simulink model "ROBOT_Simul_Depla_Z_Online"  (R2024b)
settings: Solver=ode15s  StartTime=0.0  StopTime=0.2  RelTol=1e-3  EnableMultiTasking=on
undefined symbols (not defined in the file): BATI1_Défaut_sldprt, BATI2_Défaut_sldprt, BATI3_Défaut_sldprt, BIELLE_Défaut_sldprt, BRAS_Défaut_sldprt, deg, Drive, EFFECTEUR_Défaut_sldprt, Fichiers, Fichiers_Matlab_sujetB, JOINT_Défaut_sldprt, kg, m, MANETTE_Défaut_sldprt, MATLAB, Matlab, mm, N, PIED_Défaut_sldprt, rad, s, STL, X, Y, Z
libraries: sm_lib x139, fl_lib x42, nesl_utility x19, slpidlib x3
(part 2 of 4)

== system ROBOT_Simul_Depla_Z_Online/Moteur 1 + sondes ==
  In1 : Inport
  Moteur à courant continu1 : Subsystem
  Reference electrique : fl_lib/Electrical/Electrical Elements/Electrical Reference
  Simulink-PS Converter1 : nesl_utility/Simulink-PS Converter  PhysicalDomain=network_engine_domain  SubClassName=ps_input  LeftPortType=input  RightPortType=output  PseudoPeriodic=off  Frequencies=[]  NoiseDistribution=none  NoiseParameters=[]  Unit=V  AffineConversion=off  FilteringAndDerivatives=zero  SimscapeFilterOrder=2  InputFilterTimeConstant=1e-4  UdotUserProvided=1
  Sondes électriques1 : Subsystem
  Source de tension controlée1 : fl_lib/Electrical/Electrical Sources/Controlled Voltage Source
  Conn1 : PMIOPort  Side=Right
  Conn2 : PMIOPort  Port=2  Side=Right
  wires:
  In1/1 -> Simulink-PS Converter1/1
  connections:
  Conn2/RConn1 -- Moteur à courant continu1/RConn2
  Conn1/RConn1 -- Moteur à courant continu1/RConn1
  Source de tension controlée1/LConn1 -- Sondes électriques1/LConn1
  Simulink-PS Converter1/RConn1 -- Source de tension controlée1/RConn1
  Sondes électriques1/RConn2 -- Source de tension controlée1/RConn2 -- Reference electrique/LConn1 -- Moteur à courant continu1/LConn2
  Sondes électriques1/RConn1 -- Moteur à courant continu1/LConn1

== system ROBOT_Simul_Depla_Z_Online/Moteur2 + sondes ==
  In1 : Inport
  Moteur à courant continu2 : Subsystem
  Reference electrique : fl_lib/Electrical/Electrical Elements/Electrical Reference
  Simulink-PS Converter1 : nesl_utility/Simulink-PS Converter  PhysicalDomain=network_engine_domain  SubClassName=ps_input  LeftPortType=input  RightPortType=output  PseudoPeriodic=off  Frequencies=[]  NoiseDistribution=none  NoiseParameters=[]  Unit=V  AffineConversion=off  FilteringAndDerivatives=zero  SimscapeFilterOrder=2  InputFilterTimeConstant=1e-4  UdotUserProvided=1
  Sondes électriques : Subsystem
  Source de tension controlée : fl_lib/Electrical/Electrical Sources/Controlled Voltage Source
  Conn1 : PMIOPort  Side=Right
  Conn2 : PMIOPort  Port=2  Side=Right
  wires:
  In1/1 -> Simulink-PS Converter1/1
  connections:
  Sondes électriques/RConn1 -- Moteur à courant continu2/LConn1
  Source de tension controlée/RConn2 -- Reference electrique/LConn1 -- Sondes électriques/RConn2 -- Moteur à courant continu2/LConn2
  Simulink-PS Converter1/RConn1 -- Source de tension controlée/RConn1
  Source de tension controlée/LConn1 -- Sondes électriques/LConn1
  Conn1/RConn1 -- Moteur à courant continu2/RConn1
  Conn2/RConn1 -- Moteur à courant continu2/RConn2

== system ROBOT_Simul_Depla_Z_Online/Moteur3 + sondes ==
  In1 : Inport
  Moteur à courant continu3 : Subsystem
  Reference electrique : fl_lib/Electrical/Electrical Elements/Electrical Reference
  Simulink-PS Converter1 : nesl_utility/Simulink-PS Converter  PhysicalDomain=network_engine_domain  SubClassName=ps_input  LeftPortType=input  RightPortType=output  PseudoPeriodic=off  Frequencies=[]  NoiseDistribution=none  NoiseParameters=[]  Unit=V  AffineConversion=off  FilteringAndDerivatives=zero  SimscapeFilterOrder=2  InputFilterTimeConstant=1e-4  UdotUserProvided=1
  Sondes électriques3 : Subsystem
  Source de tension controlée3 : fl_lib/Electrical/Electrical Sources/Controlled Voltage Source
  Conn1 : PMIOPort  Side=Right
  Conn2 : PMIOPort  Port=2  Side=Right
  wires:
  In1/1 -> Simulink-PS Converter1/1
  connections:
  Sondes électriques3/RConn1 -- Moteur à courant continu3/LConn1
  Moteur à courant continu3/LConn2 -- Reference electrique/LConn1 -- Source de tension controlée3/RConn2 -- Sondes électriques3/RConn2
  Simulink-PS Converter1/RConn1 -- Source de tension controlée3/RConn1
  Source de tension controlée3/LConn1 -- Sondes électriques3/LConn1
  Conn1/RConn1 -- Moteur à courant continu3/RConn1
  Conn2/RConn1 -- Moteur à courant continu3/RConn2

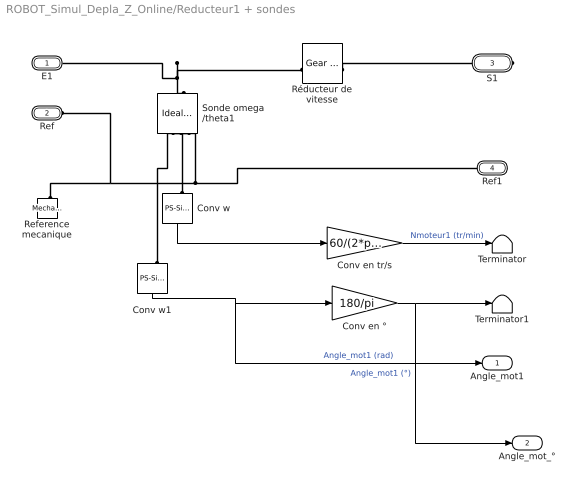
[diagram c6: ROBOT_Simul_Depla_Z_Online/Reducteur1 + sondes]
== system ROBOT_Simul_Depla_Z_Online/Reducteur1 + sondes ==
  Conv en tr/s : Gain  Gain=60/(2*pi)
  Conv en ° : Gain  Gain=180/pi
  Conv w : nesl_utility/PS-Simulink Converter  PhysicalDomain=network_engine_domain  SubClassName=ps_output  LeftPortType=input  RightPortType=output  PseudoPeriodic=off  Frequencies=[]  VectorFormat=1-D array  Unit=1  AffineConversion=off
  Conv w1 : nesl_utility/PS-Simulink Converter  PhysicalDomain=network_engine_domain  SubClassName=ps_output  LeftPortType=input  RightPortType=output  PseudoPeriodic=off  Frequencies=[]  VectorFormat=1-D array  Unit=1  AffineConversion=off
  Reference mecanique : fl_lib/Mechanical/Rotational Elements/Mechanical Rotational Reference
  Réducteur de vitesse : fl_lib/Mechanical/Mechanisms/Gear Box  ratio=7.627  t_in_specify=off  t_in_priority=None  t_in=0 N*m  t_in_nominal_specify=off  t_in_nominal_value=1  t_in_nominal_unit=N*m  t_out_specify=off  t_out_priority=None  t_out=0 N*m  t_out_nominal_specify=off  t_out_nominal_value=1  t_out_nominal_unit=N*m
  Sonde omega /theta1 : fl_lib/Mechanical/Mechanical Sensors/Ideal Rotational Motion Sensor  reference=foundation.enum.MeasurementReference.difference  acceleration_port=false  velocity_port=true  position_port=true  wrap_angle=false  offset=0 rad
  Terminator : Terminator
  Terminator1 : Terminator
  E1 : PMIOPort  Side=Left
  Ref : PMIOPort  Port=2  Side=Left
  S1 : PMIOPort  Port=3  Side=Right
  Ref1 : PMIOPort  Port=4  Side=Right
  Angle_mot1 : Outport  VectorParamsAs1DForOutWhenUnconnected=off
  Angle_mot_° : Outport  Port=2  VectorParamsAs1DForOutWhenUnconnected=off
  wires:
  Conv w1/1 -> Angle_mot1/1, Conv en °/1  "Angle_mot1 (rad)"
  Conv en °/1 -> Angle_mot_°/1, Terminator1/1  "Angle_mot1 (°)"
  Conv w/1 -> Conv en tr/s/1
  Conv en tr/s/1 -> Terminator/1  "Nmoteur1 (tr/min)"
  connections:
  Sonde omega /theta1/LConn1 -- E1/RConn1 -- Réducteur de vitesse/LConn1
  Reference mecanique/LConn1 -- Ref/RConn1 -- Sonde omega /theta1/RConn1 -- Ref1/RConn1
  Conv w/LConn1 -- Sonde omega /theta1/RConn2
  Conv w1/LConn1 -- Sonde omega /theta1/RConn3
  Réducteur de vitesse/RConn1 -- S1/RConn1

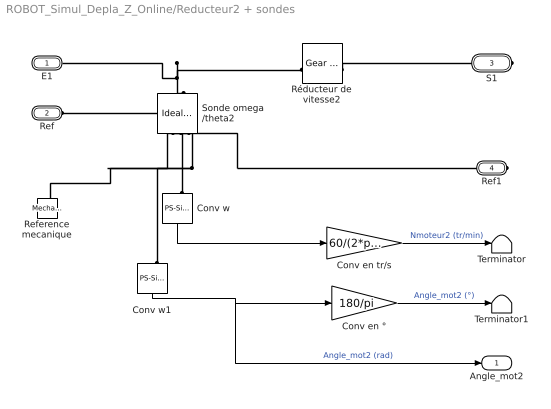
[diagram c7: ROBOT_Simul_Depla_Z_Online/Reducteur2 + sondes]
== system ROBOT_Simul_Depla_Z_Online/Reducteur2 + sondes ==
  Conv en tr/s : Gain  Gain=60/(2*pi)
  Conv en ° : Gain  Gain=180/pi
  Conv w : nesl_utility/PS-Simulink Converter  PhysicalDomain=network_engine_domain  SubClassName=ps_output  LeftPortType=input  RightPortType=output  PseudoPeriodic=off  Frequencies=[]  VectorFormat=1-D array  Unit=1  AffineConversion=off
  Conv w1 : nesl_utility/PS-Simulink Converter  PhysicalDomain=network_engine_domain  SubClassName=ps_output  LeftPortType=input  RightPortType=output  PseudoPeriodic=off  Frequencies=[]  VectorFormat=1-D array  Unit=1  AffineConversion=off
  Reference mecanique : fl_lib/Mechanical/Rotational Elements/Mechanical Rotational Reference
  Réducteur de vitesse2 : fl_lib/Mechanical/Mechanisms/Gear Box  ratio=7.627  t_in_specify=off  t_in_priority=None  t_in=0 N*m  t_in_nominal_specify=off  t_in_nominal_value=1  t_in_nominal_unit=N*m  t_out_specify=off  t_out_priority=None  t_out=0 N*m  t_out_nominal_specify=off  t_out_nominal_value=1  t_out_nominal_unit=N*m
  Sonde omega /theta2 : fl_lib/Mechanical/Mechanical Sensors/Ideal Rotational Motion Sensor  reference=foundation.enum.MeasurementReference.difference  acceleration_port=false  velocity_port=true  position_port=true  wrap_angle=false  offset=0 rad
  Terminator : Terminator
  Terminator1 : Terminator
  E1 : PMIOPort  Side=Left
  Ref : PMIOPort  Port=2  Side=Left
  S1 : PMIOPort  Port=3  Side=Right
  Ref1 : PMIOPort  Port=4  Side=Right
  Angle_mot2 : Outport  VectorParamsAs1DForOutWhenUnconnected=off
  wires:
  Conv w1/1 -> Angle_mot2/1, Conv en °/1  "Angle_mot2 (rad)"
  Conv en °/1 -> Terminator1/1  "Angle_mot2 (°)"
  Conv w/1 -> Conv en tr/s/1
  Conv en tr/s/1 -> Terminator/1  "Nmoteur2 (tr/min)"
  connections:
  Sonde omega /theta2/LConn1 -- E1/RConn1 -- Réducteur de vitesse2/LConn1
  Ref1/RConn1 -- Sonde omega /theta2/RConn1 -- Reference mecanique/LConn1 -- Ref/RConn1
  Conv w1/LConn1 -- Sonde omega /theta2/RConn3
  Conv w/LConn1 -- Sonde omega /theta2/RConn2
  Réducteur de vitesse2/RConn1 -- S1/RConn1

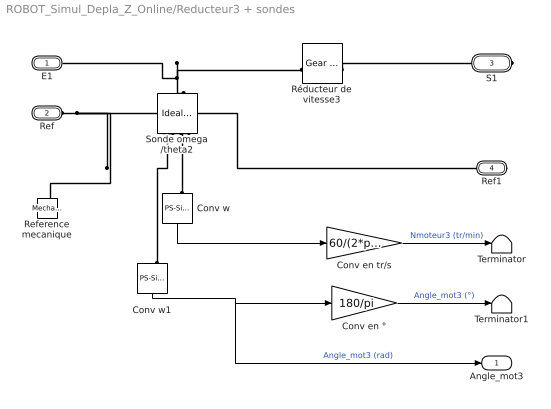
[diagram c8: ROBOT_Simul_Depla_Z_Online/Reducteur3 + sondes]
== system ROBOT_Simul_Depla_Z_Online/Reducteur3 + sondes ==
  Conv en tr/s : Gain  Gain=60/(2*pi)
  Conv en ° : Gain  Gain=180/pi
  Conv w : nesl_utility/PS-Simulink Converter  PhysicalDomain=network_engine_domain  SubClassName=ps_output  LeftPortType=input  RightPortType=output  PseudoPeriodic=off  Frequencies=[]  VectorFormat=1-D array  Unit=1  AffineConversion=off
  Conv w1 : nesl_utility/PS-Simulink Converter  PhysicalDomain=network_engine_domain  SubClassName=ps_output  LeftPortType=input  RightPortType=output  PseudoPeriodic=off  Frequencies=[]  VectorFormat=1-D array  Unit=1  AffineConversion=off
  Reference mecanique : fl_lib/Mechanical/Rotational Elements/Mechanical Rotational Reference
  Réducteur de vitesse3 : fl_lib/Mechanical/Mechanisms/Gear Box  ratio=-7.627  t_in_specify=off  t_in_priority=None  t_in=0 N*m  t_in_nominal_specify=off  t_in_nominal_value=1  t_in_nominal_unit=N*m  t_out_specify=off  t_out_priority=None  t_out=0 N*m  t_out_nominal_specify=off  t_out_nominal_value=1  t_out_nominal_unit=N*m
  Sonde omega /theta2 : fl_lib/Mechanical/Mechanical Sensors/Ideal Rotational Motion Sensor  reference=foundation.enum.MeasurementReference.difference  acceleration_port=false  velocity_port=true  position_port=true  wrap_angle=false  offset=0 rad
  Terminator : Terminator
  Terminator1 : Terminator
  E1 : PMIOPort  Side=Left
  Ref : PMIOPort  Port=2  Side=Left
  S1 : PMIOPort  Port=3  Side=Right
  Ref1 : PMIOPort  Port=4  Side=Right
  Angle_mot3 : Outport  VectorParamsAs1DForOutWhenUnconnected=off
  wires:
  Conv w1/1 -> Angle_mot3/1, Conv en °/1  "Angle_mot3 (rad)"
  Conv en °/1 -> Terminator1/1  "Angle_mot3 (°)"
  Conv w/1 -> Conv en tr/s/1
  Conv en tr/s/1 -> Terminator/1  "Nmoteur3 (tr/min)"
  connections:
  Sonde omega /theta2/LConn1 -- E1/RConn1 -- Réducteur de vitesse3/LConn1
  Ref/RConn1 -- Reference mecanique/LConn1 -- Sonde omega /theta2/RConn1 -- Ref1/RConn1
  Conv w1/LConn1 -- Sonde omega /theta2/RConn3
  Réducteur de vitesse3/RConn1 -- S1/RConn1
  Conv w/LConn1 -- Sonde omega /theta2/RConn2

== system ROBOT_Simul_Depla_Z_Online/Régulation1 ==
  In1 : Inport
  In2 : Inport  Port=2
  Add : Sum  Inputs=-+
  PID Controller : slpidlib/PID Controller  Controller=PD  Form=Parallel  TimeDomain=Continuous-time  UseExternalTs=off  SampleTime=1  IntegratorMethod=Forward Euler  FilterMethod=Forward Euler  ControllerParametersSource=internal  P=200  I=30  UseKiTs=off  D=4  UseExternalDerivativeSource=off  N=900  UseFilter=on  TunerSelectOption=Transfer Function Based (PID Tuner App)  ZeroCross=off  InitialConditionSource=internal  InitialConditionForIntegrator=0  InitialConditionForFilter=0  DifferentiatorICPrevScaledInput=0  ExternalReset=none  TrackingMode=off  Kt=1  LimitOutput=on  SatLimitsSource=internal  UpperSaturationLimit=30  LowerSaturationLimit=-30  LinearizeAsGain=off  AntiWindupMode=none  Kb=1  LimitIntegrator=off  UpperIntegratorSaturationLimit=inf  LowerIntegratorSaturationLimit=-inf  POutMin=[]  POutMax=[]  IOutMin=[]  IOutMax=[]  DOutMin=[]  DOutMax=[]  NOutMin=[]  NOutMax=[]  SumOutMin=[]  SumOutMax=[]  SaturationOutMin=[]  SaturationOutMax=[]  PParamMin=[]  PParamMax=[]  IParamMin=[]  IParamMax=[]  DParamMin=[]  DParamMax=[]  NParamMin=[]  NParamMax=[]  KbParamMin=[]  KbParamMax=[]  KtParamMin=[]  KtParamMax=[]  KbOutMin=[]  KbOutMax=[]  KtOutMin=[]  KtOutMax=[]  IntegratorOutMin=[]  IntegratorOutMax=[]  FilterOutMin=[]  FilterOutMax=[]  SumI1OutMin=[]  SumI1OutMax=[]  SumI2OutMin=[]  SumI2OutMax=[]  SumI3OutMin=[]  SumI3OutMax=[]  SumI4OutMin=[]  SumI4OutMax=[]  SumDOutMin=[]  SumDOutMax=[]  DifferentiatorOutMin=[]  DifferentiatorOutMax=[]  FilterDiffOutCoefMin=[]  FilterDiffOutCoefMax=[]  ReciprocalOutMin=[]  ReciprocalOutMax=[]  SumDenOutMin=[]  SumDenOutMax=[]  SumNumOutMin=[]  SumNumOutMax=[]  DivideOutMin=[]  DivideOutMax=[]  UdiffTsProdOutMin=[]  UdiffTsProdOutMax=[]  NTsProdOutMin=[]  NTsProdOutMax=[]  UintegralTsProdOutMin=[]  UintegralTsProdOutMax=[]  UngainTsProdOutMin=[]  UngainTsProdOutMax=[]  ClampingZeroOutDataTypeStr=Inherit: Inherit via back propagation  ClampingZeroOutMin=[]  ClampingZeroOutMax=[]  FilterDenConstantOutDataTypeStr=Inherit: Inherit via back propagation  FilterDenConstantOutMin=[]  FilterDenConstantOutMax=[]  PCopyOutDataTypeStr=Inherit: Inherit via back propagation  PCopyOutMin=[]  PCopyOutMax=[]  NCopyOutDataTypeStr=Inherit: Inherit via back propagation  NCopyOutMin=[]  NCopyOutMax=[]  IntegratorContinuousStateAttributes=''  IntegratorStateMustResolveToSignalObject=off  IntegratorRTWStateStorageClass=Auto  FilterContinuousStateAttributes=''  FilterStateMustResolveToSignalObject=off  FilterRTWStateStorageClass=Auto  ParallelPVariant=InternalParameters  IdealPVariant=Disabled  IVariant=Disabled  DVariant=InternalParameters  IntegratorVariant=Disabled  SatVariant=Enabled  AWVariant=Disabled  PCopyVariant=Disabled  TRVariant=Disabled  FdbkBlocksVariant=Forward  IdealPFdbkVariant=Disabled  SatFdbkVariant=Disabled  DerivativeFilterVariant=ContFilter  NVariant=InternalParameters  NCopyVariant=Disabled  FilterICVariant=InternalICsFilter  IntegratorICVariant=Disabled  ExternalResetVariant=Disabled  TRSumVariant=Passthrough  SumFdbkVariant=Disabled  SumVariant=Sum_PD  TsampFilterVariant=InternalTs  TsampNgainVariant=Passthrough  TsampIntegralVariant=Disabled_SignalSpec  ExternalSaturationOutDataTypeStr=Inherit: Same as second input  DerivativeSourceVariant=ErrorSignal  PreIntVariant=InternalPreInt
  Out1 : Outport  VectorParamsAs1DForOutWhenUnconnected=off
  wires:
  In1/1 -> Add/1
  In2/1 -> Add/2
  PID Controller/1 -> Out1/1
  Add/1 -> PID Controller/1

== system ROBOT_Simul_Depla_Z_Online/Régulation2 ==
  In1 : Inport
  In2 : Inport  Port=2
  Add : Sum  Inputs=-+
  PID Controller : slpidlib/PID Controller  Controller=PD  Form=Parallel  TimeDomain=Continuous-time  UseExternalTs=off  SampleTime=1  IntegratorMethod=Forward Euler  FilterMethod=Forward Euler  ControllerParametersSource=internal  P=200  I=30  UseKiTs=off  D=4  UseExternalDerivativeSource=off  N=900  UseFilter=on  TunerSelectOption=Transfer Function Based (PID Tuner App)  ZeroCross=off  InitialConditionSource=internal  InitialConditionForIntegrator=0  InitialConditionForFilter=0  DifferentiatorICPrevScaledInput=0  ExternalReset=none  TrackingMode=off  Kt=1  LimitOutput=on  SatLimitsSource=internal  UpperSaturationLimit=30  LowerSaturationLimit=-30  LinearizeAsGain=off  AntiWindupMode=none  Kb=1  LimitIntegrator=off  UpperIntegratorSaturationLimit=inf  LowerIntegratorSaturationLimit=-inf  POutMin=[]  POutMax=[]  IOutMin=[]  IOutMax=[]  DOutMin=[]  DOutMax=[]  NOutMin=[]  NOutMax=[]  SumOutMin=[]  SumOutMax=[]  SaturationOutMin=[]  SaturationOutMax=[]  PParamMin=[]  PParamMax=[]  IParamMin=[]  IParamMax=[]  DParamMin=[]  DParamMax=[]  NParamMin=[]  NParamMax=[]  KbParamMin=[]  KbParamMax=[]  KtParamMin=[]  KtParamMax=[]  KbOutMin=[]  KbOutMax=[]  KtOutMin=[]  KtOutMax=[]  IntegratorOutMin=[]  IntegratorOutMax=[]  FilterOutMin=[]  FilterOutMax=[]  SumI1OutMin=[]  SumI1OutMax=[]  SumI2OutMin=[]  SumI2OutMax=[]  SumI3OutMin=[]  SumI3OutMax=[]  SumI4OutMin=[]  SumI4OutMax=[]  SumDOutMin=[]  SumDOutMax=[]  DifferentiatorOutMin=[]  DifferentiatorOutMax=[]  FilterDiffOutCoefMin=[]  FilterDiffOutCoefMax=[]  ReciprocalOutMin=[]  ReciprocalOutMax=[]  SumDenOutMin=[]  SumDenOutMax=[]  SumNumOutMin=[]  SumNumOutMax=[]  DivideOutMin=[]  DivideOutMax=[]  UdiffTsProdOutMin=[]  UdiffTsProdOutMax=[]  NTsProdOutMin=[]  NTsProdOutMax=[]  UintegralTsProdOutMin=[]  UintegralTsProdOutMax=[]  UngainTsProdOutMin=[]  UngainTsProdOutMax=[]  ClampingZeroOutDataTypeStr=Inherit: Inherit via back propagation  ClampingZeroOutMin=[]  ClampingZeroOutMax=[]  FilterDenConstantOutDataTypeStr=Inherit: Inherit via back propagation  FilterDenConstantOutMin=[]  FilterDenConstantOutMax=[]  PCopyOutDataTypeStr=Inherit: Inherit via back propagation  PCopyOutMin=[]  PCopyOutMax=[]  NCopyOutDataTypeStr=Inherit: Inherit via back propagation  NCopyOutMin=[]  NCopyOutMax=[]  IntegratorContinuousStateAttributes=''  IntegratorStateMustResolveToSignalObject=off  IntegratorRTWStateStorageClass=Auto  FilterContinuousStateAttributes=''  FilterStateMustResolveToSignalObject=off  FilterRTWStateStorageClass=Auto  ParallelPVariant=InternalParameters  IdealPVariant=Disabled  IVariant=Disabled  DVariant=InternalParameters  IntegratorVariant=Disabled  SatVariant=Enabled  AWVariant=Disabled  PCopyVariant=Disabled  TRVariant=Disabled  FdbkBlocksVariant=Forward  IdealPFdbkVariant=Disabled  SatFdbkVariant=Disabled  DerivativeFilterVariant=ContFilter  NVariant=InternalParameters  NCopyVariant=Disabled  FilterICVariant=InternalICsFilter  IntegratorICVariant=Disabled  ExternalResetVariant=Disabled  TRSumVariant=Passthrough  SumFdbkVariant=Disabled  SumVariant=Sum_PD  TsampFilterVariant=InternalTs  TsampNgainVariant=Passthrough  TsampIntegralVariant=Disabled_SignalSpec  ExternalSaturationOutDataTypeStr=Inherit: Same as second input  DerivativeSourceVariant=ErrorSignal  PreIntVariant=InternalPreInt
  Out1 : Outport  VectorParamsAs1DForOutWhenUnconnected=off
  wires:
  Add/1 -> PID Controller/1
  PID Controller/1 -> Out1/1
  In2/1 -> Add/2
  In1/1 -> Add/1

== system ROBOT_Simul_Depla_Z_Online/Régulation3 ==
  note: Valeurs de base P=200 D=4 N=900 P=50 I=30 D=1 N=100
  In1 : Inport
  In2 : Inport  Port=2
  Add : Sum  Inputs=-+
  PID Controller : slpidlib/PID Controller  Controller=PD  Form=Parallel  TimeDomain=Continuous-time  UseExternalTs=off  SampleTime=1  IntegratorMethod=Forward Euler  FilterMethod=Forward Euler  ControllerParametersSource=internal  P=200  I=20  UseKiTs=off  D=4  UseExternalDerivativeSource=off  N=900  UseFilter=on  TunerSelectOption=Transfer Function Based (PID Tuner App)  ZeroCross=off  InitialConditionSource=internal  InitialConditionForIntegrator=0  InitialConditionForFilter=0  DifferentiatorICPrevScaledInput=0  ExternalReset=none  TrackingMode=off  Kt=1  LimitOutput=on  SatLimitsSource=internal  UpperSaturationLimit=30  LowerSaturationLimit=-30  LinearizeAsGain=off  AntiWindupMode=none  Kb=1  LimitIntegrator=off  UpperIntegratorSaturationLimit=inf  LowerIntegratorSaturationLimit=-inf  POutMin=[]  POutMax=[]  IOutMin=[]  IOutMax=[]  DOutMin=[]  DOutMax=[]  NOutMin=[]  NOutMax=[]  SumOutMin=[]  SumOutMax=[]  SaturationOutMin=[]  SaturationOutMax=[]  PParamMin=[]  PParamMax=[]  IParamMin=[]  IParamMax=[]  DParamMin=[]  DParamMax=[]  NParamMin=[]  NParamMax=[]  KbParamMin=[]  KbParamMax=[]  KtParamMin=[]  KtParamMax=[]  KbOutMin=[]  KbOutMax=[]  KtOutMin=[]  KtOutMax=[]  IntegratorOutMin=[]  IntegratorOutMax=[]  FilterOutMin=[]  FilterOutMax=[]  SumI1OutMin=[]  SumI1OutMax=[]  SumI2OutMin=[]  SumI2OutMax=[]  SumI3OutMin=[]  SumI3OutMax=[]  SumI4OutMin=[]  SumI4OutMax=[]  SumDOutMin=[]  SumDOutMax=[]  DifferentiatorOutMin=[]  DifferentiatorOutMax=[]  FilterDiffOutCoefMin=[]  FilterDiffOutCoefMax=[]  ReciprocalOutMin=[]  ReciprocalOutMax=[]  SumDenOutMin=[]  SumDenOutMax=[]  SumNumOutMin=[]  SumNumOutMax=[]  DivideOutMin=[]  DivideOutMax=[]  UdiffTsProdOutMin=[]  UdiffTsProdOutMax=[]  NTsProdOutMin=[]  NTsProdOutMax=[]  UintegralTsProdOutMin=[]  UintegralTsProdOutMax=[]  UngainTsProdOutMin=[]  UngainTsProdOutMax=[]  ClampingZeroOutDataTypeStr=Inherit: Inherit via back propagation  ClampingZeroOutMin=[]  ClampingZeroOutMax=[]  FilterDenConstantOutDataTypeStr=Inherit: Inherit via back propagation  FilterDenConstantOutMin=[]  FilterDenConstantOutMax=[]  PCopyOutDataTypeStr=Inherit: Inherit via back propagation  PCopyOutMin=[]  PCopyOutMax=[]  NCopyOutDataTypeStr=Inherit: Inherit via back propagation  NCopyOutMin=[]  NCopyOutMax=[]  IntegratorContinuousStateAttributes=''  IntegratorStateMustResolveToSignalObject=off  IntegratorRTWStateStorageClass=Auto  FilterContinuousStateAttributes=''  FilterStateMustResolveToSignalObject=off  FilterRTWStateStorageClass=Auto  ParallelPVariant=InternalParameters  IdealPVariant=Disabled  IVariant=Disabled  DVariant=InternalParameters  IntegratorVariant=Disabled  SatVariant=Enabled  AWVariant=Disabled  PCopyVariant=Disabled  TRVariant=Disabled  FdbkBlocksVariant=Forward  IdealPFdbkVariant=Disabled  SatFdbkVariant=Disabled  DerivativeFilterVariant=ContFilter  NVariant=InternalParameters  NCopyVariant=Disabled  FilterICVariant=InternalICsFilter  IntegratorICVariant=Disabled  ExternalResetVariant=Disabled  TRSumVariant=Passthrough  SumFdbkVariant=Disabled  SumVariant=Sum_PD  TsampFilterVariant=InternalTs  TsampNgainVariant=Passthrough  TsampIntegralVariant=Disabled_SignalSpec  ExternalSaturationOutDataTypeStr=Inherit: Same as second input  DerivativeSourceVariant=ErrorSignal  PreIntVariant=InternalPreInt
  Out1 : Outport  VectorParamsAs1DForOutWhenUnconnected=off
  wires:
  Add/1 -> PID Controller/1
  PID Controller/1 -> Out1/1
  In2/1 -> Add/2
  In1/1 -> Add/1

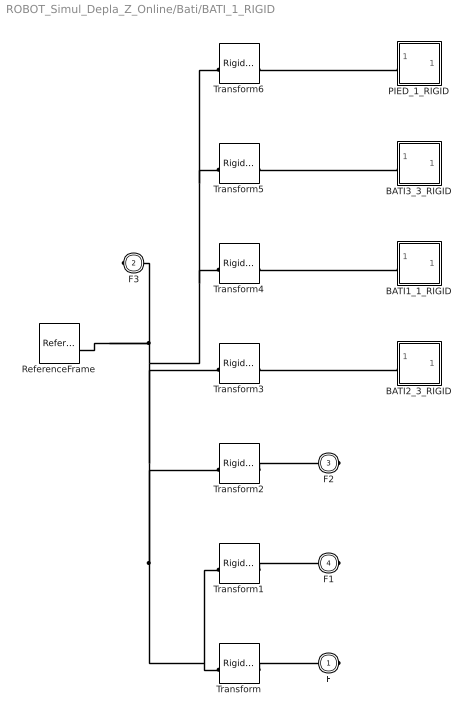
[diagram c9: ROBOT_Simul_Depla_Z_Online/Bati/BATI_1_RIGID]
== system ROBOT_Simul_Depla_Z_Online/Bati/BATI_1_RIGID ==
  BATI1_1_RIGID : Subsystem
  BATI2_3_RIGID : Subsystem
  BATI3_3_RIGID : Subsystem
  PIED_1_RIGID : Subsystem
  ReferenceFrame : sm_lib/Frames and Transforms/Reference Frame
  Transform : sm_lib/Frames and Transforms/Rigid Transform  RotationMethod=ArbitraryAxis  FollAlignAxisA=+X  BaseAlignAxisA=+Y  FollAlignAxisB=+Y  BaseAlignAxisB=+Z  RotationStandardAxis=+Z  RotationAngle=2.0943951023931953  RotationAngleUnits=rad  RotationArbitraryAxis=[-0.57735026918962584 -0.57735026918962584 0.57735026918962584]  RotationSequenceAxes=FollowerAxes  RotationSequence=XYX  RotationSequenceAngles=[0 0 0]  RotationSequenceAnglesUnits=deg  RotationMatrix=[1 0 0; 0 1 0; 0 0 1]  Quaternion=[1 0 0 0]  TranslationMethod=Cartesian  TranslationCartesianOffset=[11.464585537616552 15.162590585005695 19.999999999988876]  TranslationCartesianOffsetUnits=mm  TranslationStandardAxis=+Z  TranslationStandardOffset=0  TranslationStandardOffsetUnits=mm  TranslationROffset=0  TranslationROffsetUnits=m  TranslationThetaOffset=0  TranslationThetaOffsetUnits=deg  TranslationZOffset=0  TranslationZOffsetUnits=m
  Transform1 : sm_lib/Frames and Transforms/Rigid Transform  RotationMethod=ArbitraryAxis  FollAlignAxisA=+X  BaseAlignAxisA=+Y  FollAlignAxisB=+Y  BaseAlignAxisB=+Z  RotationStandardAxis=+Z  RotationAngle=2.4188584057763811  RotationAngleUnits=rad  RotationArbitraryAxis=[0.65465367070797764 -0.37796447300922537 0.65465367070797764]  RotationSequenceAxes=FollowerAxes  RotationSequence=XYX  RotationSequenceAngles=[0 0 0]  RotationSequenceAnglesUnits=deg  RotationMatrix=[1 0 0; 0 1 0; 0 0 1]  Quaternion=[1 0 0 0]  TranslationMethod=Cartesian  TranslationCartesianOffset=[-74.272540245284446 -12.683808110643664 19.999999999988628]  TranslationCartesianOffsetUnits=mm  TranslationStandardAxis=+Z  TranslationStandardOffset=0  TranslationStandardOffsetUnits=mm  TranslationROffset=0  TranslationROffsetUnits=m  TranslationThetaOffset=0  TranslationThetaOffsetUnits=deg  TranslationZOffset=0  TranslationZOffsetUnits=m
  Transform2 : sm_lib/Frames and Transforms/Rigid Transform  RotationMethod=ArbitraryAxis  FollAlignAxisA=+X  BaseAlignAxisA=+Y  FollAlignAxisB=+Y  BaseAlignAxisB=+Z  RotationStandardAxis=+Z  RotationAngle=2.4188584057763713  RotationAngleUnits=rad  RotationArbitraryAxis=[-0.65465367070797609 -0.37796447300923092 -0.65465367070797609]  RotationSequenceAxes=FollowerAxes  RotationSequence=XYX  RotationSequenceAngles=[0 0 0]  RotationSequenceAnglesUnits=deg  RotationMatrix=[1 0 0; 0 1 0; 0 0 1]  Quaternion=[1 0 0 0]  TranslationMethod=Cartesian  TranslationCartesianOffset=[-9.7882886794943111 -68.68101071934548 19.999999999988635]  TranslationCartesianOffsetUnits=mm  TranslationStandardAxis=+Z  TranslationStandardOffset=0  TranslationStandardOffsetUnits=mm  TranslationROffset=0  TranslationROffsetUnits=m  TranslationThetaOffset=0  TranslationThetaOffsetUnits=deg  TranslationZOffset=0  TranslationZOffsetUnits=m
  Transform3 : sm_lib/Frames and Transforms/Rigid Transform  RotationMethod=None  FollAlignAxisA=+X  BaseAlignAxisA=+Y  FollAlignAxisB=+Y  BaseAlignAxisB=+Z  RotationStandardAxis=+Z  RotationAngle=0  RotationAngleUnits=deg  RotationArbitraryAxis=[0 0 1]  RotationSequenceAxes=FollowerAxes  RotationSequence=XYX  RotationSequenceAngles=[0 0 0]  RotationSequenceAnglesUnits=deg  RotationMatrix=[1 0 0; 0 1 0; 0 0 1]  Quaternion=[1 0 0 0]  TranslationMethod=Cartesian  TranslationCartesianOffset=[-25.865414462389737 -22.06740941499433 -1.1369377661551994e-11]  TranslationCartesianOffsetUnits=mm  TranslationStandardAxis=+Z  TranslationStandardOffset=0  TranslationStandardOffsetUnits=mm  TranslationROffset=0  TranslationROffsetUnits=m  TranslationThetaOffset=0  TranslationThetaOffsetUnits=deg  TranslationZOffset=0  TranslationZOffsetUnits=m
  Transform4 : sm_lib/Frames and Transforms/Rigid Transform  RotationMethod=ArbitraryAxis  FollAlignAxisA=+X  BaseAlignAxisA=+Y  FollAlignAxisB=+Y  BaseAlignAxisB=+Z  RotationStandardAxis=+Z  RotationAngle=2.0943951023932001  RotationAngleUnits=rad  RotationArbitraryAxis=[0 0 1]  RotationSequenceAxes=FollowerAxes  RotationSequence=XYX  RotationSequenceAngles=[0 0 0]  RotationSequenceAnglesUnits=deg  RotationMatrix=[1 0 0; 0 1 0; 0 0 1]  Quaternion=[1 0 0 0]  TranslationMethod=Cartesian  TranslationCartesianOffset=[-25.865414462389737 -22.06740941499433 -1.136590821460004e-11]  TranslationCartesianOffsetUnits=mm  TranslationStandardAxis=+Z  TranslationStandardOffset=0  TranslationStandardOffsetUnits=mm  TranslationROffset=0  TranslationROffsetUnits=m  TranslationThetaOffset=0  TranslationThetaOffsetUnits=deg  TranslationZOffset=0  TranslationZOffsetUnits=m
  Transform5 : sm_lib/Frames and Transforms/Rigid Transform  RotationMethod=ArbitraryAxis  FollAlignAxisA=+X  BaseAlignAxisA=+Y  FollAlignAxisB=+Y  BaseAlignAxisB=+Z  RotationStandardAxis=+Z  RotationAngle=2.0943951023931855  RotationAngleUnits=rad  RotationArbitraryAxis=[-0 -0 -1]  RotationSequenceAxes=FollowerAxes  RotationSequence=XYX  RotationSequenceAngles=[0 0 0]  RotationSequenceAnglesUnits=deg  RotationMatrix=[1 0 0; 0 1 0; 0 0 1]  Quaternion=[1 0 0 0]  TranslationMethod=Cartesian  TranslationCartesianOffset=[-25.86541446238942 -22.06740941499471 -1.136590821460004e-11]  TranslationCartesianOffsetUnits=mm  TranslationStandardAxis=+Z  TranslationStandardOffset=0  TranslationStandardOffsetUnits=mm  TranslationROffset=0  TranslationROffsetUnits=m  TranslationThetaOffset=0  TranslationThetaOffsetUnits=deg  TranslationZOffset=0  TranslationZOffsetUnits=m
  Transform6 : sm_lib/Frames and Transforms/Rigid Transform  RotationMethod=ArbitraryAxis  FollAlignAxisA=+X  BaseAlignAxisA=+Y  FollAlignAxisB=+Y  BaseAlignAxisB=+Z  RotationStandardAxis=+Z  RotationAngle=2.0943951023932006  RotationAngleUnits=rad  RotationArbitraryAxis=[0 0 1]  RotationSequenceAxes=FollowerAxes  RotationSequence=XYX  RotationSequenceAngles=[0 0 0]  RotationSequenceAnglesUnits=deg  RotationMatrix=[1 0 0; 0 1 0; 0 0 1]  Quaternion=[1 0 0 0]  TranslationMethod=Cartesian  TranslationCartesianOffset=[-25.865414462390763 -22.06740941499276 9.9999999999886313]  TranslationCartesianOffsetUnits=mm  TranslationStandardAxis=+Z  TranslationStandardOffset=0  TranslationStandardOffsetUnits=mm  TranslationROffset=0  TranslationROffsetUnits=m  TranslationThetaOffset=0  TranslationThetaOffsetUnits=deg  TranslationZOffset=0  TranslationZOffsetUnits=m
  F : PMIOPort  Side=Right
  F3 : PMIOPort  Port=2  Side=Left
  F2 : PMIOPort  Port=3  Side=Right
  F1 : PMIOPort  Port=4  Side=Right
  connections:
  Transform/LConn1 -- Transform5/LConn1 -- Transform6/LConn1 -- Transform4/LConn1 -- ReferenceFrame/RConn1 -- F3/RConn1 -- Transform3/LConn1 -- Transform2/LConn1 -- Transform1/LConn1
  Transform/RConn1 -- F/RConn1
  Transform1/RConn1 -- F1/RConn1
  Transform2/RConn1 -- F2/RConn1
  BATI2_3_RIGID/LConn1 -- Transform3/RConn1
  BATI1_1_RIGID/LConn1 -- Transform4/RConn1
  BATI3_3_RIGID/LConn1 -- Transform5/RConn1
  PIED_1_RIGID/LConn1 -- Transform6/RConn1

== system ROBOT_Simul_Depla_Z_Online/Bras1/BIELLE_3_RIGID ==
  ReferenceFrame : sm_lib/Frames and Transforms/Reference Frame
  Solid : sm_lib/Body Elements/File Solid  ExtGeomFileName=/MATLAB Drive/Fichiers_Matlab_sujetB/Fichiers Matlab/STL/BIELLE_Défaut_sldprt.STL  UnitType=Custom  ExtGeomFileUnits=mm  StepReaderType=HEX  ExportConvexHullGeometry=off  InertiaType=Custom  BasedOnType=Density  Density=1000  DensityUnits=kg/(m^3)  Mass=0.008350539405564527  MassUnits=kg  CenterOfMass=[0 1.3968069938607398e-07 -5.4963035279888423e-06]  CenterOfMassUnits=mm  MomentsOfInertia=[9.7237898508136684 9.7147278737202658 0.035523108889582884]  MomentsOfInertiaUnits=kg*mm^2  ProductsOfInertia=[0 -4.4011490170351759e-08 -8.1673382975267321e-07]  ProductsOfInertiaUnits=kg*mm^2  GraphicType=FromGeometry  MarkerShape=Sphere  MarkerSize=10  GraphicVisPropType=SimpleVisualProperties  GraphicDiffuseColor=[0.69803921568627447 0.69803921568627447 0.69803921568627447]  GraphicOpacity=1  GraphicSpecularColor=[0.5 0.5 0.5 1.0]  GraphicAmbientColor=[0.15 0.15 0.15 1.0]  GraphicEmissiveColor=[0.0 0.0 0.0 1.0]  GraphicShininess=75  DoExposeReferenceFrame=on  SerializedFrames=<Frames/>
  Transform : sm_lib/Frames and Transforms/Rigid Transform  RotationMethod=ArbitraryAxis  FollAlignAxisA=+X  BaseAlignAxisA=+Y  FollAlignAxisB=+Y  BaseAlignAxisB=+Z  RotationStandardAxis=+Z  RotationAngle=2.0943951023931957  RotationAngleUnits=rad  RotationArbitraryAxis=[0.57735026918962584 -0.57735026918962573 0.57735026918962573]  RotationSequenceAxes=FollowerAxes  RotationSequence=XYX  RotationSequenceAngles=[0 0 0]  RotationSequenceAnglesUnits=deg  RotationMatrix=[1 0 0; 0 1 0; 0 0 1]  Quaternion=[1 0 0 0]  TranslationMethod=Cartesian  TranslationCartesianOffset=[0 4.9999999999999902 -51.25]  TranslationCartesianOffsetUnits=mm  TranslationStandardAxis=+Z  TranslationStandardOffset=0  TranslationStandardOffsetUnits=mm  TranslationROffset=0  TranslationROffsetUnits=m  TranslationThetaOffset=0  TranslationThetaOffsetUnits=deg  TranslationZOffset=0  TranslationZOffsetUnits=m
  Transform1 : sm_lib/Frames and Transforms/Rigid Transform  RotationMethod=ArbitraryAxis  FollAlignAxisA=+X  BaseAlignAxisA=+Y  FollAlignAxisB=+Y  BaseAlignAxisB=+Z  RotationStandardAxis=+Z  RotationAngle=2.0943951023931957  RotationAngleUnits=rad  RotationArbitraryAxis=[0.57735026918962584 -0.57735026918962573 0.57735026918962573]  RotationSequenceAxes=FollowerAxes  RotationSequence=XYX  RotationSequenceAngles=[0 0 0]  RotationSequenceAnglesUnits=deg  RotationMatrix=[1 0 0; 0 1 0; 0 0 1]  Quaternion=[1 0 0 0]  TranslationMethod=Cartesian  TranslationCartesianOffset=[0 4.9999999999999769 51.249999999999986]  TranslationCartesianOffsetUnits=mm  TranslationStandardAxis=+Z  TranslationStandardOffset=0  TranslationStandardOffsetUnits=mm  TranslationROffset=0  TranslationROffsetUnits=m  TranslationThetaOffset=0  TranslationThetaOffsetUnits=deg  TranslationZOffset=0  TranslationZOffsetUnits=m
  F1 : PMIOPort  Side=Left
  F : PMIOPort  Port=2  Side=Right
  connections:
  Solid/RConn1 -- ReferenceFrame/RConn1 -- Transform/LConn1 -- Transform1/LConn1
  Transform/RConn1 -- F/RConn1
  Transform1/RConn1 -- F1/RConn1

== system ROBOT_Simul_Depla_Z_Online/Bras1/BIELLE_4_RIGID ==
  ReferenceFrame : sm_lib/Frames and Transforms/Reference Frame
  Solid : sm_lib/Body Elements/File Solid  ExtGeomFileName=/MATLAB Drive/Fichiers_Matlab_sujetB/Fichiers Matlab/STL/BIELLE_Défaut_sldprt.STL  UnitType=Custom  ExtGeomFileUnits=mm  StepReaderType=HEX  ExportConvexHullGeometry=off  InertiaType=Custom  BasedOnType=Density  Density=1000  DensityUnits=kg/(m^3)  Mass=0.008350539405564527  MassUnits=kg  CenterOfMass=[0 1.3968069938607398e-07 -5.4963035279888423e-06]  CenterOfMassUnits=mm  MomentsOfInertia=[9.7237898508136684 9.7147278737202658 0.035523108889582884]  MomentsOfInertiaUnits=kg*mm^2  ProductsOfInertia=[0 -4.4011490170351759e-08 -8.1673382975267321e-07]  ProductsOfInertiaUnits=kg*mm^2  GraphicType=FromGeometry  MarkerShape=Sphere  MarkerSize=10  GraphicVisPropType=SimpleVisualProperties  GraphicDiffuseColor=[0.69803921568627447 0.69803921568627447 0.69803921568627447]  GraphicOpacity=1  GraphicSpecularColor=[0.5 0.5 0.5 1.0]  GraphicAmbientColor=[0.15 0.15 0.15 1.0]  GraphicEmissiveColor=[0.0 0.0 0.0 1.0]  GraphicShininess=75  DoExposeReferenceFrame=on  SerializedFrames=<Frames/>
  Transform : sm_lib/Frames and Transforms/Rigid Transform  RotationMethod=ArbitraryAxis  FollAlignAxisA=+X  BaseAlignAxisA=+Y  FollAlignAxisB=+Y  BaseAlignAxisB=+Z  RotationStandardAxis=+Z  RotationAngle=2.0943951023931953  RotationAngleUnits=rad  RotationArbitraryAxis=[0.57735026918962584 -0.57735026918962584 0.57735026918962584]  RotationSequenceAxes=FollowerAxes  RotationSequence=XYX  RotationSequenceAngles=[0 0 0]  RotationSequenceAnglesUnits=deg  RotationMatrix=[1 0 0; 0 1 0; 0 0 1]  Quaternion=[1 0 0 0]  TranslationMethod=Cartesian  TranslationCartesianOffset=[0 4.9999999999999902 -51.250000000000014]  TranslationCartesianOffsetUnits=mm  TranslationStandardAxis=+Z  TranslationStandardOffset=0  TranslationStandardOffsetUnits=mm  TranslationROffset=0  TranslationROffsetUnits=m  TranslationThetaOffset=0  TranslationThetaOffsetUnits=deg  TranslationZOffset=0  TranslationZOffsetUnits=m
  Transform1 : sm_lib/Frames and Transforms/Rigid Transform  RotationMethod=ArbitraryAxis  FollAlignAxisA=+X  BaseAlignAxisA=+Y  FollAlignAxisB=+Y  BaseAlignAxisB=+Z  RotationStandardAxis=+Z  RotationAngle=2.0943951023931953  RotationAngleUnits=rad  RotationArbitraryAxis=[0.57735026918962584 -0.57735026918962584 0.57735026918962584]  RotationSequenceAxes=FollowerAxes  RotationSequence=XYX  RotationSequenceAngles=[0 0 0]  RotationSequenceAnglesUnits=deg  RotationMatrix=[1 0 0; 0 1 0; 0 0 1]  Quaternion=[1 0 0 0]  TranslationMethod=Cartesian  TranslationCartesianOffset=[0 5.0000000000000044 51.250000000000014]  TranslationCartesianOffsetUnits=mm  TranslationStandardAxis=+Z  TranslationStandardOffset=0  TranslationStandardOffsetUnits=mm  TranslationROffset=0  TranslationROffsetUnits=m  TranslationThetaOffset=0  TranslationThetaOffsetUnits=deg  TranslationZOffset=0  TranslationZOffsetUnits=m
  F1 : PMIOPort  Side=Left
  F : PMIOPort  Port=2  Side=Right
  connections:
  Solid/RConn1 -- ReferenceFrame/RConn1 -- Transform/LConn1 -- Transform1/LConn1
  Transform/RConn1 -- F/RConn1
  Transform1/RConn1 -- F1/RConn1

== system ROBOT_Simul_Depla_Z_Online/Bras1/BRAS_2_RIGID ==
  BRAS_1_RIGID : Subsystem
  BRAS_3_RIGID : Subsystem
  ReferenceFrame : sm_lib/Frames and Transforms/Reference Frame
  Transform : sm_lib/Frames and Transforms/Rigid Transform  RotationMethod=ArbitraryAxis  FollAlignAxisA=+X  BaseAlignAxisA=+Y  FollAlignAxisB=+Y  BaseAlignAxisB=+Z  RotationStandardAxis=+Z  RotationAngle=1.852259063952334e-15  RotationAngleUnits=rad  RotationArbitraryAxis=[-0.27659366947124742 0.96098696245497017 -2.4616792487648572e-16]  RotationSequenceAxes=FollowerAxes  RotationSequence=XYX  RotationSequenceAngles=[0 0 0]  RotationSequenceAnglesUnits=deg  RotationMatrix=[1 0 0; 0 1 0; 0 0 1]  Quaternion=[1 0 0 0]  TranslationMethod=Cartesian  TranslationCartesianOffset=[-9.6989083431253675e-13 -16.842456388464441 -5.0000000000000027]  TranslationCartesianOffsetUnits=mm  TranslationStandardAxis=+Z  TranslationStandardOffset=0  TranslationStandardOffsetUnits=mm  TranslationROffset=0  TranslationROffsetUnits=m  TranslationThetaOffset=0  TranslationThetaOffsetUnits=deg  TranslationZOffset=0  TranslationZOffsetUnits=m
  Transform1 : sm_lib/Frames and Transforms/Rigid Transform  RotationMethod=ArbitraryAxis  FollAlignAxisA=+X  BaseAlignAxisA=+Y  FollAlignAxisB=+Y  BaseAlignAxisB=+Z  RotationStandardAxis=+Z  RotationAngle=3.1415926535897931  RotationAngleUnits=rad  RotationArbitraryAxis=[1 0 0]  RotationSequenceAxes=FollowerAxes  RotationSequence=XYX  RotationSequenceAngles=[0 0 0]  RotationSequenceAnglesUnits=deg  RotationMatrix=[1 0 0; 0 1 0; 0 0 1]  Quaternion=[1 0 0 0]  TranslationMethod=Cartesian  TranslationCartesianOffset=[0 43.157543611535324 10.000000000006278]  TranslationCartesianOffsetUnits=mm  TranslationStandardAxis=+Z  TranslationStandardOffset=0  TranslationStandardOffsetUnits=mm  TranslationROffset=0  TranslationROffsetUnits=m  TranslationThetaOffset=0  TranslationThetaOffsetUnits=deg  TranslationZOffset=0  TranslationZOffsetUnits=m
  Transform2 : sm_lib/Frames and Transforms/Rigid Transform  RotationMethod=None  FollAlignAxisA=+X  BaseAlignAxisA=+Y  FollAlignAxisB=+Y  BaseAlignAxisB=+Z  RotationStandardAxis=+Z  RotationAngle=0  RotationAngleUnits=deg  RotationArbitraryAxis=[0 0 1]  RotationSequenceAxes=FollowerAxes  RotationSequence=XYX  RotationSequenceAngles=[0 0 0]  RotationSequenceAnglesUnits=deg  RotationMatrix=[1 0 0; 0 1 0; 0 0 1]  Quaternion=[1 0 0 0]  TranslationMethod=Cartesian  TranslationCartesianOffset=[0 -16.842456388464662 6.2727600891321345e-12]  TranslationCartesianOffsetUnits=mm  TranslationStandardAxis=+Z  TranslationStandardOffset=0  TranslationStandardOffsetUnits=mm  TranslationROffset=0  TranslationROffsetUnits=m  TranslationThetaOffset=0  TranslationThetaOffsetUnits=deg  TranslationZOffset=0  TranslationZOffsetUnits=m
  Transform3 : sm_lib/Frames and Transforms/Rigid Transform  RotationMethod=ArbitraryAxis  FollAlignAxisA=+X  BaseAlignAxisA=+Y  FollAlignAxisB=+Y  BaseAlignAxisB=+Z  RotationStandardAxis=+Z  RotationAngle=3.1415926535897931  RotationAngleUnits=rad  RotationArbitraryAxis=[0 0 1]  RotationSequenceAxes=FollowerAxes  RotationSequence=XYX  RotationSequenceAngles=[0 0 0]  RotationSequenceAnglesUnits=deg  RotationMatrix=[1 0 0; 0 1 0; 0 0 1]  Quaternion=[1 0 0 0]  TranslationMethod=Cartesian  TranslationCartesianOffset=[0 43.157543611535324 6.2796989830360417e-12]  TranslationCartesianOffsetUnits=mm  TranslationStandardAxis=+Z  TranslationStandardOffset=0  TranslationStandardOffsetUnits=mm  TranslationROffset=0  TranslationROffsetUnits=m  TranslationThetaOffset=0  TranslationThetaOffsetUnits=deg  TranslationZOffset=0  TranslationZOffsetUnits=m
  F : PMIOPort  Side=Left
  F1 : PMIOPort  Port=2  Side=Right
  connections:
  Transform/LConn1 -- ReferenceFrame/RConn1 -- Transform1/LConn1 -- Transform2/LConn1 -- Transform3/LConn1
  Transform/RConn1 -- F/RConn1
  Transform1/RConn1 -- F1/RConn1
  BRAS_1_RIGID/LConn1 -- Transform2/RConn1
  BRAS_3_RIGID/LConn1 -- Transform3/RConn1

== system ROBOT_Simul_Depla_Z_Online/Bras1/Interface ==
  Angular Velocity Source : fl_lib/Mechanical/Mechanical Sources/Ideal Angular Velocity Source
  Torque Sensor : fl_lib/Mechanical/Mechanical Sensors/Ideal Torque Sensor
  C : PMIOPort  Side=Left
  T : PMIOPort  Port=2  Side=Right
  w : PMIOPort  Port=3  Side=Right
  R : PMIOPort  Port=4  Side=Left
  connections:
  R/RConn1 -- Angular Velocity Source/LConn1
  Torque Sensor/LConn1 -- Angular Velocity Source/RConn2
  Torque Sensor/RConn2 -- T/RConn1
  C/RConn1 -- Torque Sensor/RConn1
  Angular Velocity Source/RConn1 -- w/RConn1

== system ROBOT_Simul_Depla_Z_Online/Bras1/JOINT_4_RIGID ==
  ReferenceFrame : sm_lib/Frames and Transforms/Reference Frame
  Solid : sm_lib/Body Elements/File Solid  ExtGeomFileName=/MATLAB Drive/Fichiers_Matlab_sujetB/Fichiers Matlab/STL/JOINT_Défaut_sldprt.STL  UnitType=Custom  ExtGeomFileUnits=mm  StepReaderType=HEX  ExportConvexHullGeometry=off  InertiaType=Custom  BasedOnType=Density  Density=1000  DensityUnits=kg/(m^3)  Mass=0.010425088409650831  MassUnits=kg  CenterOfMass=[-2.8413803884081348e-07 7.2198924235006832 8.2870434049836507e-08]  CenterOfMassUnits=mm  MomentsOfInertia=[0.40441054898779027 0.67355736496231777 0.88349580308055875]  MomentsOfInertiaUnits=kg*mm^2  ProductsOfInertia=[5.448486796310623e-10 1.7393207622030534e-07 1.1975376403711247e-08]  ProductsOfInertiaUnits=kg*mm^2  GraphicType=FromGeometry  MarkerShape=Sphere  MarkerSize=10  GraphicVisPropType=SimpleVisualProperties  GraphicDiffuseColor=[0.792156862745098 0.81960784313725488 0.93333333333333335]  GraphicOpacity=1  GraphicSpecularColor=[0.5 0.5 0.5 1.0]  GraphicAmbientColor=[0.15 0.15 0.15 1.0]  GraphicEmissiveColor=[0.0 0.0 0.0 1.0]  GraphicShininess=75  DoExposeReferenceFrame=on  SerializedFrames=<Frames/>
  Transform : sm_lib/Frames and Transforms/Rigid Transform  RotationMethod=ArbitraryAxis  FollAlignAxisA=+X  BaseAlignAxisA=+Y  FollAlignAxisB=+Y  BaseAlignAxisB=+Z  RotationStandardAxis=+Z  RotationAngle=3.1415926535897931  RotationAngleUnits=rad  RotationArbitraryAxis=[-1 4.2709310989463294e-33 -8.8869701386798953e-17]  RotationSequenceAxes=FollowerAxes  RotationSequence=XYX  RotationSequenceAngles=[0 0 0]  RotationSequenceAnglesUnits=deg  RotationMatrix=[1 0 0; 0 1 0; 0 0 1]  Quaternion=[1 0 0 0]  TranslationMethod=Cartesian  TranslationCartesianOffset=[13.999999999999849 4.9999999999999574 4.9999999999999956]  TranslationCartesianOffsetUnits=mm  TranslationStandardAxis=+Z  TranslationStandardOffset=0  TranslationStandardOffsetUnits=mm  TranslationROffset=0  TranslationROffsetUnits=m  TranslationThetaOffset=0  TranslationThetaOffsetUnits=deg  TranslationZOffset=0  TranslationZOffsetUnits=m
  Transform1 : sm_lib/Frames and Transforms/Rigid Transform  RotationMethod=ArbitraryAxis  FollAlignAxisA=+X  BaseAlignAxisA=+Y  FollAlignAxisB=+Y  BaseAlignAxisB=+Z  RotationStandardAxis=+Z  RotationAngle=1.5700924586837749e-16  RotationAngleUnits=rad  RotationArbitraryAxis=[-0.99993539825238109 0.011366587959979699 -8.9227205578830452e-19]  RotationSequenceAxes=FollowerAxes  RotationSequence=XYX  RotationSequenceAngles=[0 0 0]  RotationSequenceAnglesUnits=deg  RotationMatrix=[1 0 0; 0 1 0; 0 0 1]  Quaternion=[1 0 0 0]  TranslationMethod=Cartesian  TranslationCartesianOffset=[-14.000000000000142 4.9999999999998455 -4.9999999999999893]  TranslationCartesianOffsetUnits=mm  TranslationStandardAxis=+Z  TranslationStandardOffset=0  TranslationStandardOffsetUnits=mm  TranslationROffset=0  TranslationROffsetUnits=m  TranslationThetaOffset=0  TranslationThetaOffsetUnits=deg  TranslationZOffset=0  TranslationZOffsetUnits=m
  Transform2 : sm_lib/Frames and Transforms/Rigid Transform  RotationMethod=ArbitraryAxis  FollAlignAxisA=+X  BaseAlignAxisA=+Y  FollAlignAxisB=+Y  BaseAlignAxisB=+Z  RotationStandardAxis=+Z  RotationAngle=2.0943951023931944  RotationAngleUnits=rad  RotationArbitraryAxis=[0.57735026918962729 0.57735026918962551 0.57735026918962451]  RotationSequenceAxes=FollowerAxes  RotationSequence=XYX  RotationSequenceAngles=[0 0 0]  RotationSequenceAnglesUnits=deg  RotationMatrix=[1 0 0; 0 1 0; 0 0 1]  Quaternion=[1 0 0 0]  TranslationMethod=Cartesian  TranslationCartesianOffset=[-9.9999999999997335 16.250000000000529 -3.0198066269804258e-13]  TranslationCartesianOffsetUnits=mm  TranslationStandardAxis=+Z  TranslationStandardOffset=0  TranslationStandardOffsetUnits=mm  TranslationROffset=0  TranslationROffsetUnits=m  TranslationThetaOffset=0  TranslationThetaOffsetUnits=deg  TranslationZOffset=0  TranslationZOffsetUnits=m
  F2 : PMIOPort  Side=Right
  F1 : PMIOPort  Port=2  Side=Left
  F : PMIOPort  Port=3  Side=Left
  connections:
  Solid/RConn1 -- ReferenceFrame/RConn1 -- Transform1/LConn1 -- Transform2/LConn1 -- Transform/LConn1
  Transform/RConn1 -- F/RConn1
  Transform1/RConn1 -- F1/RConn1
  Transform2/RConn1 -- F2/RConn1

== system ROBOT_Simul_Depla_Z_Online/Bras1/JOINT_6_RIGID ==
  ReferenceFrame : sm_lib/Frames and Transforms/Reference Frame
  Solid : sm_lib/Body Elements/File Solid  ExtGeomFileName=/MATLAB Drive/Fichiers_Matlab_sujetB/Fichiers Matlab/STL/JOINT_Défaut_sldprt.STL  UnitType=Custom  ExtGeomFileUnits=mm  StepReaderType=HEX  ExportConvexHullGeometry=off  InertiaType=Custom  BasedOnType=Density  Density=1000  DensityUnits=kg/(m^3)  Mass=0.010425088409650831  MassUnits=kg  CenterOfMass=[-2.8413803884081348e-07 7.2198924235006832 8.2870434049836507e-08]  CenterOfMassUnits=mm  MomentsOfInertia=[0.40441054898779027 0.67355736496231777 0.88349580308055875]  MomentsOfInertiaUnits=kg*mm^2  ProductsOfInertia=[5.448486796310623e-10 1.7393207622030534e-07 1.1975376403711247e-08]  ProductsOfInertiaUnits=kg*mm^2  GraphicType=FromGeometry  MarkerShape=Sphere  MarkerSize=10  GraphicVisPropType=SimpleVisualProperties  GraphicDiffuseColor=[0.792156862745098 0.81960784313725488 0.93333333333333335]  GraphicOpacity=1  GraphicSpecularColor=[0.5 0.5 0.5 1.0]  GraphicAmbientColor=[0.15 0.15 0.15 1.0]  GraphicEmissiveColor=[0.0 0.0 0.0 1.0]  GraphicShininess=75  DoExposeReferenceFrame=on  SerializedFrames=<Frames/>
  Transform : sm_lib/Frames and Transforms/Rigid Transform  RotationMethod=ArbitraryAxis  FollAlignAxisA=+X  BaseAlignAxisA=+Y  FollAlignAxisB=+Y  BaseAlignAxisB=+Z  RotationStandardAxis=+Z  RotationAngle=2.5476231888929306e-16  RotationAngleUnits=rad  RotationArbitraryAxis=[0.25866689172319263 0.96596658282068038 3.1827911693718406e-17]  RotationSequenceAxes=FollowerAxes  RotationSequence=XYX  RotationSequenceAngles=[0 0 0]  RotationSequenceAnglesUnits=deg  RotationMatrix=[1 0 0; 0 1 0; 0 0 1]  Quaternion=[1 0 0 0]  TranslationMethod=Cartesian  TranslationCartesianOffset=[14.000000000000327 5.0000000000000409 -4.9999999999999645]  TranslationCartesianOffsetUnits=mm  TranslationStandardAxis=+Z  TranslationStandardOffset=0  TranslationStandardOffsetUnits=mm  TranslationROffset=0  TranslationROffsetUnits=m  TranslationThetaOffset=0  TranslationThetaOffsetUnits=deg  TranslationZOffset=0  TranslationZOffsetUnits=m
  Transform1 : sm_lib/Frames and Transforms/Rigid Transform  RotationMethod=ArbitraryAxis  FollAlignAxisA=+X  BaseAlignAxisA=+Y  FollAlignAxisB=+Y  BaseAlignAxisB=+Z  RotationStandardAxis=+Z  RotationAngle=3.1415926535897931  RotationAngleUnits=rad  RotationArbitraryAxis=[1 -6.1548272841853811e-33 -8.2569214265266672e-17]  RotationSequenceAxes=FollowerAxes  RotationSequence=XYX  RotationSequenceAngles=[0 0 0]  RotationSequenceAnglesUnits=deg  RotationMatrix=[1 0 0; 0 1 0; 0 0 1]  Quaternion=[1 0 0 0]  TranslationMethod=Cartesian  TranslationCartesianOffset=[-13.999999999999677 5.0000000000000444 4.9999999999999964]  TranslationCartesianOffsetUnits=mm  TranslationStandardAxis=+Z  TranslationStandardOffset=0  TranslationStandardOffsetUnits=mm  TranslationROffset=0  TranslationROffsetUnits=m  TranslationThetaOffset=0  TranslationThetaOffsetUnits=deg  TranslationZOffset=0  TranslationZOffsetUnits=m
  Transform2 : sm_lib/Frames and Transforms/Rigid Transform  RotationMethod=ArbitraryAxis  FollAlignAxisA=+X  BaseAlignAxisA=+Y  FollAlignAxisB=+Y  BaseAlignAxisB=+Z  RotationStandardAxis=+Z  RotationAngle=2.0943951023931966  RotationAngleUnits=rad  RotationArbitraryAxis=[-0.5773502691896264 -0.57735026918962618 0.57735026918962484]  RotationSequenceAxes=FollowerAxes  RotationSequence=XYX  RotationSequenceAngles=[0 0 0]  RotationSequenceAnglesUnits=deg  RotationMatrix=[1 0 0; 0 1 0; 0 0 1]  Quaternion=[1 0 0 0]  TranslationMethod=Cartesian  TranslationCartesianOffset=[10.000000000006413 16.249999999997939 -2.3288038164537284e-12]  TranslationCartesianOffsetUnits=mm  TranslationStandardAxis=+Z  TranslationStandardOffset=0  TranslationStandardOffsetUnits=mm  TranslationROffset=0  TranslationROffsetUnits=m  TranslationThetaOffset=0  TranslationThetaOffsetUnits=deg  TranslationZOffset=0  TranslationZOffsetUnits=m
  F2 : PMIOPort  Side=Left
  F1 : PMIOPort  Port=2  Side=Right
  F : PMIOPort  Port=3  Side=Right
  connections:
  Solid/RConn1 -- ReferenceFrame/RConn1 -- Transform1/LConn1 -- Transform2/LConn1 -- Transform/LConn1
  Transform/RConn1 -- F/RConn1
  Transform1/RConn1 -- F1/RConn1
  Transform2/RConn1 -- F2/RConn1
